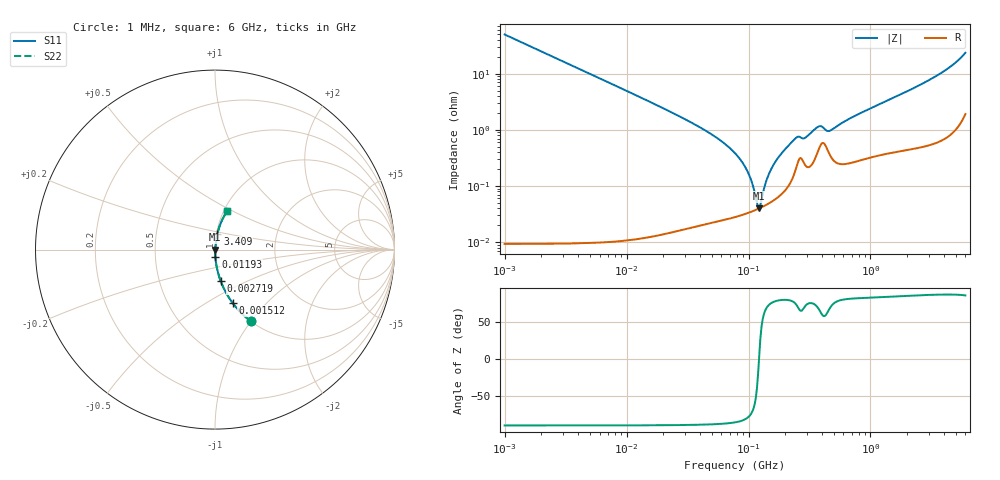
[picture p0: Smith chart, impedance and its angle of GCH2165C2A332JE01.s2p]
!Murata Part Number: GCH2165C2A332JE01
!These Parameters are Measured in Series Mode Connection
!Data Generated on Jun 19, 2026
!  o--ll--o
!Port1  Port2
!  o------o
!Operation Temp=25[degC], DC Bias Voltage=0[V]
!Freq. Start=1000[kHz] Stop=6[GHz] 401[Steps]
# Hz S RI R 50
!Freq.(Hz) S11(Real) S11(Imag) S21(Real) S21(Imag) S12(Real) S12(Imag) S22(Real) S22(Imag)
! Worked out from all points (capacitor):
!   401 points, 1 MHz to 6 GHz, reference 50 ohm
!   read as one part in series: C = 3.2 nF near 1.044 MHz
!   lowest |Z| = 40 mohm at 122.3 MHz (marker M1)
!   series resonance near 121.9 MHz, so ESL is about 530 pH
!   S11 on the Smith chart (normalised r, x): 1 MHz: 1.00, -1.00; 1.512 MHz: 1.00, -0.66; 2.719 MHz: 1.00, -0.37; 11.93 MHz: 1.00, -0.08; 3.409 GHz: 1.01, +0.18; 6 GHz: 1.04, +0.47
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1000000  0.1985 -0.3987  0.8015 0.3987  0.8015 0.3987  0.1985 -0.3987
1511688  0.0978 -0.2969  0.9022 0.2969  0.9022 0.2969  0.0978 -0.2969
2719490  0.0324 -0.1769  0.9676 0.1769  0.9676 0.1769  0.0324 -0.1769
4293785  0.0133 -0.1142  0.9867 0.1142  0.9867 0.1142  0.0133 -0.1142
1.193364e7  0.00181 -0.0412  0.9982 0.0412  0.9982 0.0412  0.00181 -0.0412
1.843659e7  0.000825 -0.0263  0.9992 0.0263  0.9992 0.0263  0.000825 -0.0263
4.697123e7  0.000294 -0.00898  0.9997 0.00898  0.9997 0.00898  0.000294 -0.00898
7.745967e7  0.000294 -0.00382  0.9997 0.00382  0.9997 0.00382  0.000294 -0.00382
9.83954e7  0.000332 -0.00176  0.9997 0.00176  0.9997 0.00176  0.000332 -0.00176
1.073387e8  0.000355 -0.00104  0.9996 0.00104  0.9996 0.00104  0.000355 -0.00104
1.170949e8  0.000382 -0.00033  0.9996 0.00033  0.9996 0.00033  0.000382 -0.00033
1.223006e8  0.000399 2.7e-05  0.9996 -2.7e-05  0.9996 -2.7e-05  0.000399 2.7e-05
1.455431e8  0.000487 0.00148  0.9995 -0.00148  0.9995 -0.00148  0.000487 0.00148
1.732027e8  0.000632 0.00302  0.9994 -0.00302  0.9994 -0.00302  0.000632 0.00302
2.452905e8  0.00211 0.00685  0.9979 -0.00685  0.9979 -0.00685  0.00211 0.00685
2.919064e8  0.00237 0.00679  0.9976 -0.00679  0.9976 -0.00679  0.00237 0.00679
3.325952e8  0.00253 0.00893  0.9975 -0.00893  0.9975 -0.00893  0.00253 0.00893
3.872876e8  0.00526 0.0103  0.9947 -0.0103  0.9947 -0.0103  0.00526 0.0103
4.710229e8  0.00345 0.0091  0.9966 -0.0091  0.9966 -0.0091  0.00345 0.0091
1.428092e9  0.00495 0.0338  0.995 -0.0338  0.995 -0.0338  0.00495 0.0338
3.408564e9  0.0134 0.0872  0.9866 -0.0872  0.9866 -0.0872  0.0134 0.0872
6e9  0.0681 0.2145  0.9319 -0.2145  0.9319 -0.2145  0.0681 0.2145
